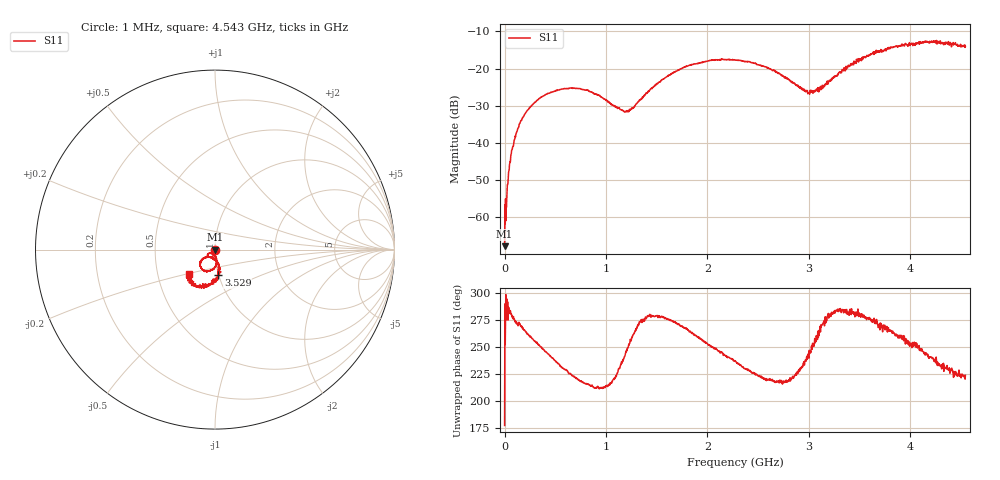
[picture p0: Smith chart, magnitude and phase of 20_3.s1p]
# HZ S RI R 50
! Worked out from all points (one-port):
!   1515 points, 1 MHz to 4.543 GHz, reference 50 ohm
!   lowest |S11| = -67.8 dB at 1 MHz (marker M1), VSWR 1.00, Z = 50 + j0.0021 ohm
!   |S11| at or under -10 dB: start of sweep to end of sweep
!   S11 on the Smith chart (normalised r, x): 1 MHz: 1.00, +0.00; 3.529 GHz: 1.00, -0.29; 4.543 GHz: 0.72, -0.21
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1000000  -0.000409 2.11e-05
1.3e7  0.000427 -0.000792
2.5e7  0.00021 -0.00216
4.6e7  0.000866 -0.00424
5.8e7  0.00128 -0.00542
9.1e7  0.00103 -0.00993
1.45e8  0.000688 -0.0177
2.26e8  -0.00369 -0.0271
3.4e8  -0.0125 -0.0374
5.71e8  -0.0337 -0.041
8.23e8  -0.0412 -0.0294
1.138e9  -0.0181 -0.0216
1.198e9  -0.0109 -0.0242
1.246e9  -0.00725 -0.0274
1.483e9  0.00807 -0.058
1.705e9  0.00226 -0.0936
2.029e9  -0.0428 -0.1215
2.272e9  -0.0724 -0.1092
2.578e9  -0.0795 -0.0677
2.842e9  -0.0468 -0.0431
2.986e9  -0.024 -0.0445
3.061e9  -0.0133 -0.0472
3.409e9  0.0277 -0.1058
3.529e9  0.0187 -0.1414
3.793e9  -0.0186 -0.1877
3.976e9  -0.0494 -0.1927
4.237e9  -0.1208 -0.1945
4.543e9  -0.1439 -0.1363
